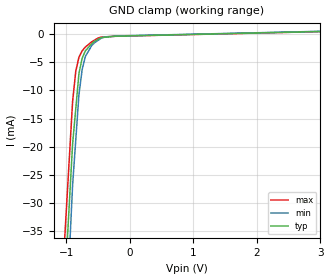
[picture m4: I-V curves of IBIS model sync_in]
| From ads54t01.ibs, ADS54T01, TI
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[Model] sync_in
Model_type Input
Vinl = 1.12500V
Vinh = 1.37500V
C_comp 596.000fF 574.000fF 618.000fF
| variable typ   min   max
[Voltage Range] 1.80000V 1.65000V 1.95000V
[POWER Clamp Reference] 1.80000V 1.65000V 1.95000V
[GND Clamp Reference] 0.00000V 0.00000V 0.00000V
[Temperature Range]   25   85   -40
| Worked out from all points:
|   GND clamp passes 1 mA (typ) near -0.51 V on its own axis
[GND Clamp]
-1.8V     -204.7mA   -240.8mA   -188.1mA
-900mV    -19.53mA   -26.85mA   -11.99mA
-850mV    -13.27mA   -18.8mA    -6.61mA
-800mV    -7.008mA   -10.75mA   -4.108mA
-750mV    -4.312mA   -6.33mA    -2.986mA
-700mV    -3.002mA   -3.993mA   -2.318mA
-600mV    -1.722mA   -2.065mA   -1.394mA
-500mV    -951uA     -1.125mA   -717uA
-450mV    -636.1uA   -746uA     -533.4uA
-400mV    -579.3uA   -525.1uA   -503uA
-200mV    -373.7uA   -337.6uA   -390.2uA
3.6V      615.1uA    639.4uA    583.7uA
[POWER Clamp]
-1.8V     0A         0A         0A
3.6V      0A         0A         0A
